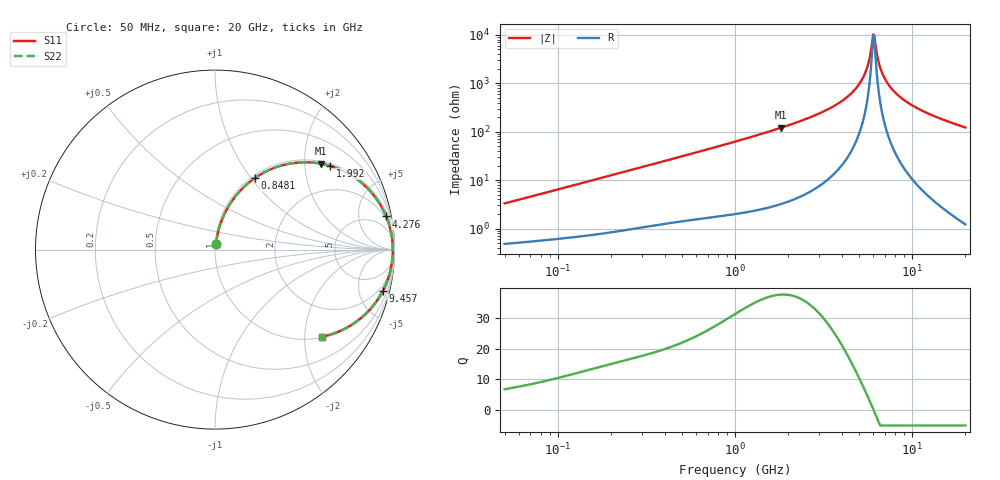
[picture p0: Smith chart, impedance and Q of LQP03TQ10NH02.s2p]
!Murata Part Number: LQP03TQ10NH02
!These Parameters are Measured in Series Mode Connection
!  o--[Z]--o
!Port1  Port2
!  o-------o
!Freq. Start=50[MHz] Stop=20[GHz], 401[Steps]
# Hz S RI R 50
!Freq.(Hz) S11(Real) S11(Imag) S21(Real) S21(Imag) S12(Real) S12(Imag) S22(Real) S22(Imag)
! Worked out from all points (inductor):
!   401 points, 50 MHz to 20 GHz, reference 50 ohm
!   read as one part in series: L = 10.3 nH near 51.52 MHz
!   highest Q = 37.6 at 1.821 GHz (marker M1), where L = 10.5 nH
!   self-resonance near 6.034 GHz
!   S11 on the Smith chart (normalised r, x): 50 MHz: 1.01, +0.07; 848.1 MHz: 1.04, +1.05; 1.992 GHz: 1.07, +2.69; 4.276 GHz: 2, +10; 9.457 GHz: 1.27, -7.96; 20 GHz: 1.02, -2.44
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5e7  0.00585 0.0323  0.9941 -0.0323  0.9941 -0.0323  0.00585 0.0323
1.364002e8  0.0142 0.0848  0.9858 -0.0848  0.9858 -0.0848  0.0142 0.0848
3.721004e8  0.0608 0.2143  0.9392 -0.2143  0.9392 -0.2143  0.0608 0.2143
8.480927e8  0.2243 0.4001  0.7757 -0.4001  0.7757 -0.4001  0.2243 0.4001
1e9  0.2858 0.4361  0.7142 -0.4361  0.7142 -0.4361  0.2858 0.4361
1.820564e9  0.5907 0.4786  0.4093 -0.4786  0.4093 -0.4786  0.5907 0.4786
1.99176e9  0.6409 0.4666  0.3591 -0.4666  0.3591 -0.4666  0.6409 0.4666
2.728004e9  0.8023 0.3837  0.1977 -0.3837  0.1977 -0.3837  0.8023 0.3837
3.519108e9  0.902 0.2789  0.098 -0.2789  0.098 -0.2789  0.902 0.2789
4.275624e9  0.9538 0.1844  0.0462 -0.1844  0.0462 -0.1844  0.9538 0.1844
4.81993e9  0.9746 0.1226  0.0254 -0.1226  0.0254 -0.1226  0.9746 0.1226
5.273168e9  0.9846 0.0751  0.0154 -0.0751  0.0154 -0.0751  0.9846 0.0751
5.598765e9  0.9886 0.0431  0.0114 -0.0431  0.0114 -0.0431  0.9886 0.0431
5.944466e9  0.9906 0.011  0.00945 -0.011  0.00945 -0.011  0.9906 0.011
6.034176e9  0.9907 0.00292  0.00929 -0.00292  0.00929 -0.00292  0.9907 0.00292
6.217679e9  0.9906 -0.0132  0.00939 0.0132  0.00939 0.0132  0.9906 -0.0132
6.503449e9  0.9895 -0.0373  0.0105 0.0373  0.0105 0.0373  0.9895 -0.0373
6.701223e9  0.9881 -0.0534  0.0119 0.0534  0.0119 0.0534  0.9881 -0.0534
7.442007e9  0.979 -0.1092  0.021 0.1092  0.021 0.1092  0.979 -0.1092
9.457416e9  0.9336 -0.2324  0.0664 0.2324  0.0664 0.2324  0.9336 -0.2324
1.314879e10  0.8167 -0.3781  0.1833 0.3781  0.1833 0.3781  0.8167 -0.3781
2e10  0.5974 -0.4854  0.4026 0.4854  0.4026 0.4854  0.5974 -0.4854
